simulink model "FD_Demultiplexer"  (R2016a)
settings: Solver=ode3  StartTime=0.0  StopTime=6  FixedStep=1/5000000  RelTol=1e-3
libraries: dsparch4 x4, commsynccomp2 x4, simulink x4

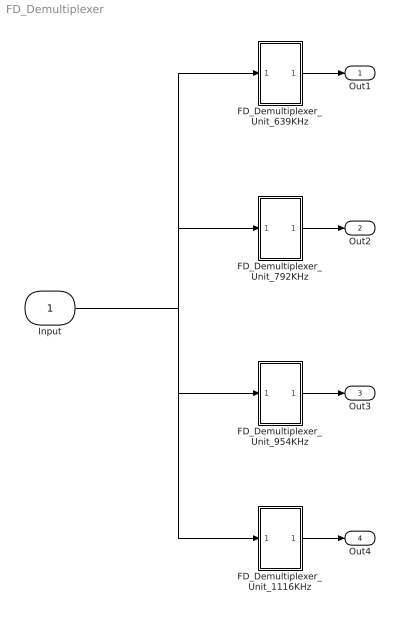
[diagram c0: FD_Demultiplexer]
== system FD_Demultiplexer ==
  Input : Inport
  FD_Demultiplexer_Unit_1116KHz : Subsystem
  FD_Demultiplexer_Unit_639KHz : Subsystem
  FD_Demultiplexer_Unit_792KHz : Subsystem
  FD_Demultiplexer_Unit_954KHz : Subsystem
  Out1 : Outport
  Out2 : Outport  Port=2
  Out3 : Outport  Port=3
  Out4 : Outport  Port=4
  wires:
  Input/1 -> FD_Demultiplexer_Unit_1116KHz/1(In1), FD_Demultiplexer_Unit_954KHz/1(In1), FD_Demultiplexer_Unit_792KHz/1(In1), FD_Demultiplexer_Unit_639KHz/1(In1)
  FD_Demultiplexer_Unit_639KHz/1(Out1) -> Out1/1
  FD_Demultiplexer_Unit_792KHz/1(Out1) -> Out2/1
  FD_Demultiplexer_Unit_954KHz/1(Out1) -> Out3/1
  FD_Demultiplexer_Unit_1116KHz/1(Out1) -> Out4/1

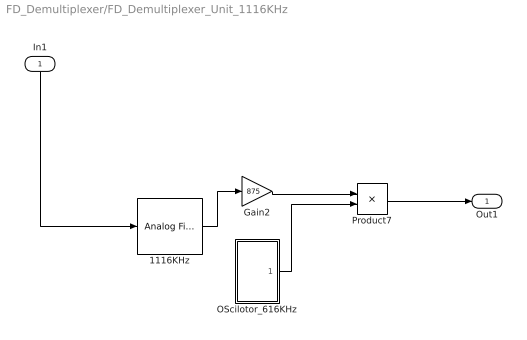
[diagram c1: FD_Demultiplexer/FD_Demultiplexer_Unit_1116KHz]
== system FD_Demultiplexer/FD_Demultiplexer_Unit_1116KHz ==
  In1 : Inport
  1116KHz : dsparch4/Analog Filter Design  method=Butterworth  filttype=Bandpass  N=8  Wlo=1066000*2*pi  Whi=1166000*2*pi  Rp=2  Rs=60
  Gain2 : Gain  Gain=875
  OScilotor_616KHz : Subsystem
  Product7 : Product
  Out1 : Outport
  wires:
  1116KHz/1 -> Gain2/1
  Product7/1 -> Out1/1
  Gain2/1 -> Product7/1
  OScilotor_616KHz/1(Output) -> Product7/2
  In1/1 -> 1116KHz/1

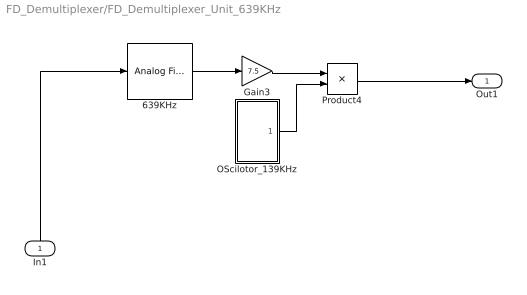
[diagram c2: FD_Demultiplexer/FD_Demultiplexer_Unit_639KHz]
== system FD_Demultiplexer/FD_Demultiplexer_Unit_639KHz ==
  In1 : Inport
  639KHz : dsparch4/Analog Filter Design  method=Butterworth  filttype=Bandpass  N=8  Wlo=589000*2*pi  Whi=689000*2*pi  Rp=2  Rs=40
  Gain3 : Gain  Gain=7.5
  OScilotor_139KHz : Subsystem
  Product4 : Product
  Out1 : Outport
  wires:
  Product4/1 -> Out1/1
  639KHz/1 -> Gain3/1
  OScilotor_139KHz/1(Output) -> Product4/2
  Gain3/1 -> Product4/1
  In1/1 -> 639KHz/1

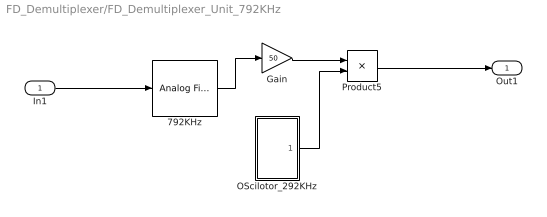
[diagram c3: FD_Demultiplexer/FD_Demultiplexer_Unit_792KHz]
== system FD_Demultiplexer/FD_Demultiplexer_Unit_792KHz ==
  In1 : Inport
  792KHz : dsparch4/Analog Filter Design  method=Butterworth  filttype=Bandpass  N=8  Wlo=742000*2*pi  Whi=842000*2*pi  Rp=2  Rs=40
  Gain : Gain  Gain=50
  OScilotor_292KHz : Subsystem
  Product5 : Product
  Out1 : Outport
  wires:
  Product5/1 -> Out1/1
  Gain/1 -> Product5/1
  792KHz/1 -> Gain/1
  OScilotor_292KHz/1(Output) -> Product5/2
  In1/1 -> 792KHz/1

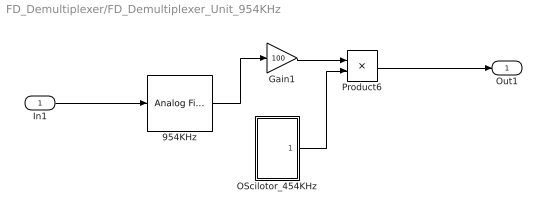
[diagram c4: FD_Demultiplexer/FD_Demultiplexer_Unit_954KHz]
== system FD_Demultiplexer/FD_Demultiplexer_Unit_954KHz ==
  In1 : Inport
  954KHz : dsparch4/Analog Filter Design  method=Butterworth  filttype=Bandpass  N=8  Wlo=904000*2*pi  Whi=1004000*2*pi  Rp=2  Rs=40
  Gain1 : Gain  Gain=100
  OScilotor_454KHz : Subsystem
  Product6 : Product
  Out1 : Outport
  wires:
  OScilotor_454KHz/1(Output) -> Product6/2
  Product6/1 -> Out1/1
  954KHz/1 -> Gain1/1
  Gain1/1 -> Product6/1
  In1/1 -> 954KHz/1

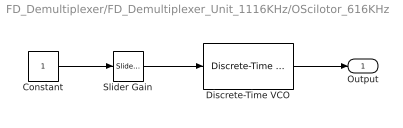
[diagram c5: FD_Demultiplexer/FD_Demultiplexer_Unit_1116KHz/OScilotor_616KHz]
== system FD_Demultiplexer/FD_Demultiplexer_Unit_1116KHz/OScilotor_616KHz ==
  Constant : Constant
  Discrete-Time VCO : commsynccomp2/Discrete-Time VCO  Ac=1  Fc=0  Kc=1000  Ph=0  ts=1/5000000
  Slider Gain : simulink/Math Operations/Slider Gain  low=616  gain=616  high=2070
  Output : Outport
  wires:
  Constant/1 -> Slider Gain/1
  Slider Gain/1 -> Discrete-Time VCO/1
  Discrete-Time VCO/1 -> Output/1

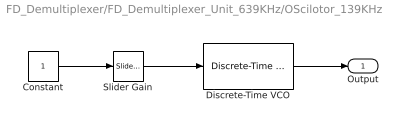
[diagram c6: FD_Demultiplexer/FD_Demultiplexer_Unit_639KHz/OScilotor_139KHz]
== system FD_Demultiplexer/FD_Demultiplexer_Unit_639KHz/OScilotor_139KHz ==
  Constant : Constant
  Discrete-Time VCO : commsynccomp2/Discrete-Time VCO  Ac=1  Fc=0  Kc=1000  Ph=0  ts=1/5000000
  Slider Gain : simulink/Math Operations/Slider Gain  low=139  gain=139  high=2070
  Output : Outport
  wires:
  Constant/1 -> Slider Gain/1
  Slider Gain/1 -> Discrete-Time VCO/1
  Discrete-Time VCO/1 -> Output/1

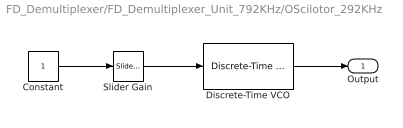
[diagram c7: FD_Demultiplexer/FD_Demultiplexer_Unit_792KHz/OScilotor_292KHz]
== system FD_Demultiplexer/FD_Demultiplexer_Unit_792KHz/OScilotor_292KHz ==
  Constant : Constant
  Discrete-Time VCO : commsynccomp2/Discrete-Time VCO  Ac=1  Fc=0  Kc=1000  Ph=0  ts=1/5000000
  Slider Gain : simulink/Math Operations/Slider Gain  low=292  gain=292  high=2070
  Output : Outport
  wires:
  Constant/1 -> Slider Gain/1
  Slider Gain/1 -> Discrete-Time VCO/1
  Discrete-Time VCO/1 -> Output/1

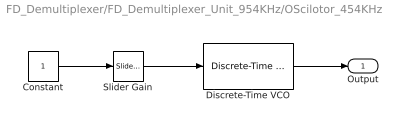
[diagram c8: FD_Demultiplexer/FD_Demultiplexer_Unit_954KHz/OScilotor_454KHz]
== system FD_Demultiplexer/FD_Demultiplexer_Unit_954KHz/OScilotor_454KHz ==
  Constant : Constant
  Discrete-Time VCO : commsynccomp2/Discrete-Time VCO  Ac=1  Fc=0  Kc=1000  Ph=0  ts=1/5000000
  Slider Gain : simulink/Math Operations/Slider Gain  low=454  gain=454  high=2070
  Output : Outport
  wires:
  Constant/1 -> Slider Gain/1
  Slider Gain/1 -> Discrete-Time VCO/1
  Discrete-Time VCO/1 -> Output/1
